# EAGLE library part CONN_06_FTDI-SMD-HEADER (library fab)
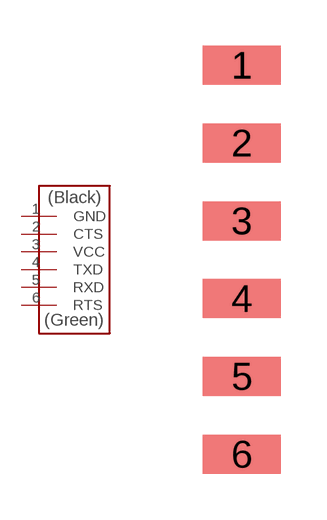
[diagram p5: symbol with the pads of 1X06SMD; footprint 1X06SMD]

Designator prefix -

## CONN_06_FTDI-SMD-HEADER  [1X06SMD]
1  GND
2  CTS
3  VCC
4  TXD
5  RXD
6  RTS

## Footprint 1X06SMD (pad centres in mm)
smd 2.54 x 1.27: 1 0,6.35; 2 0,3.81; 3 0,1.27; 4 0,-1.27; 5 0,-3.81; 6 0,-6.35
